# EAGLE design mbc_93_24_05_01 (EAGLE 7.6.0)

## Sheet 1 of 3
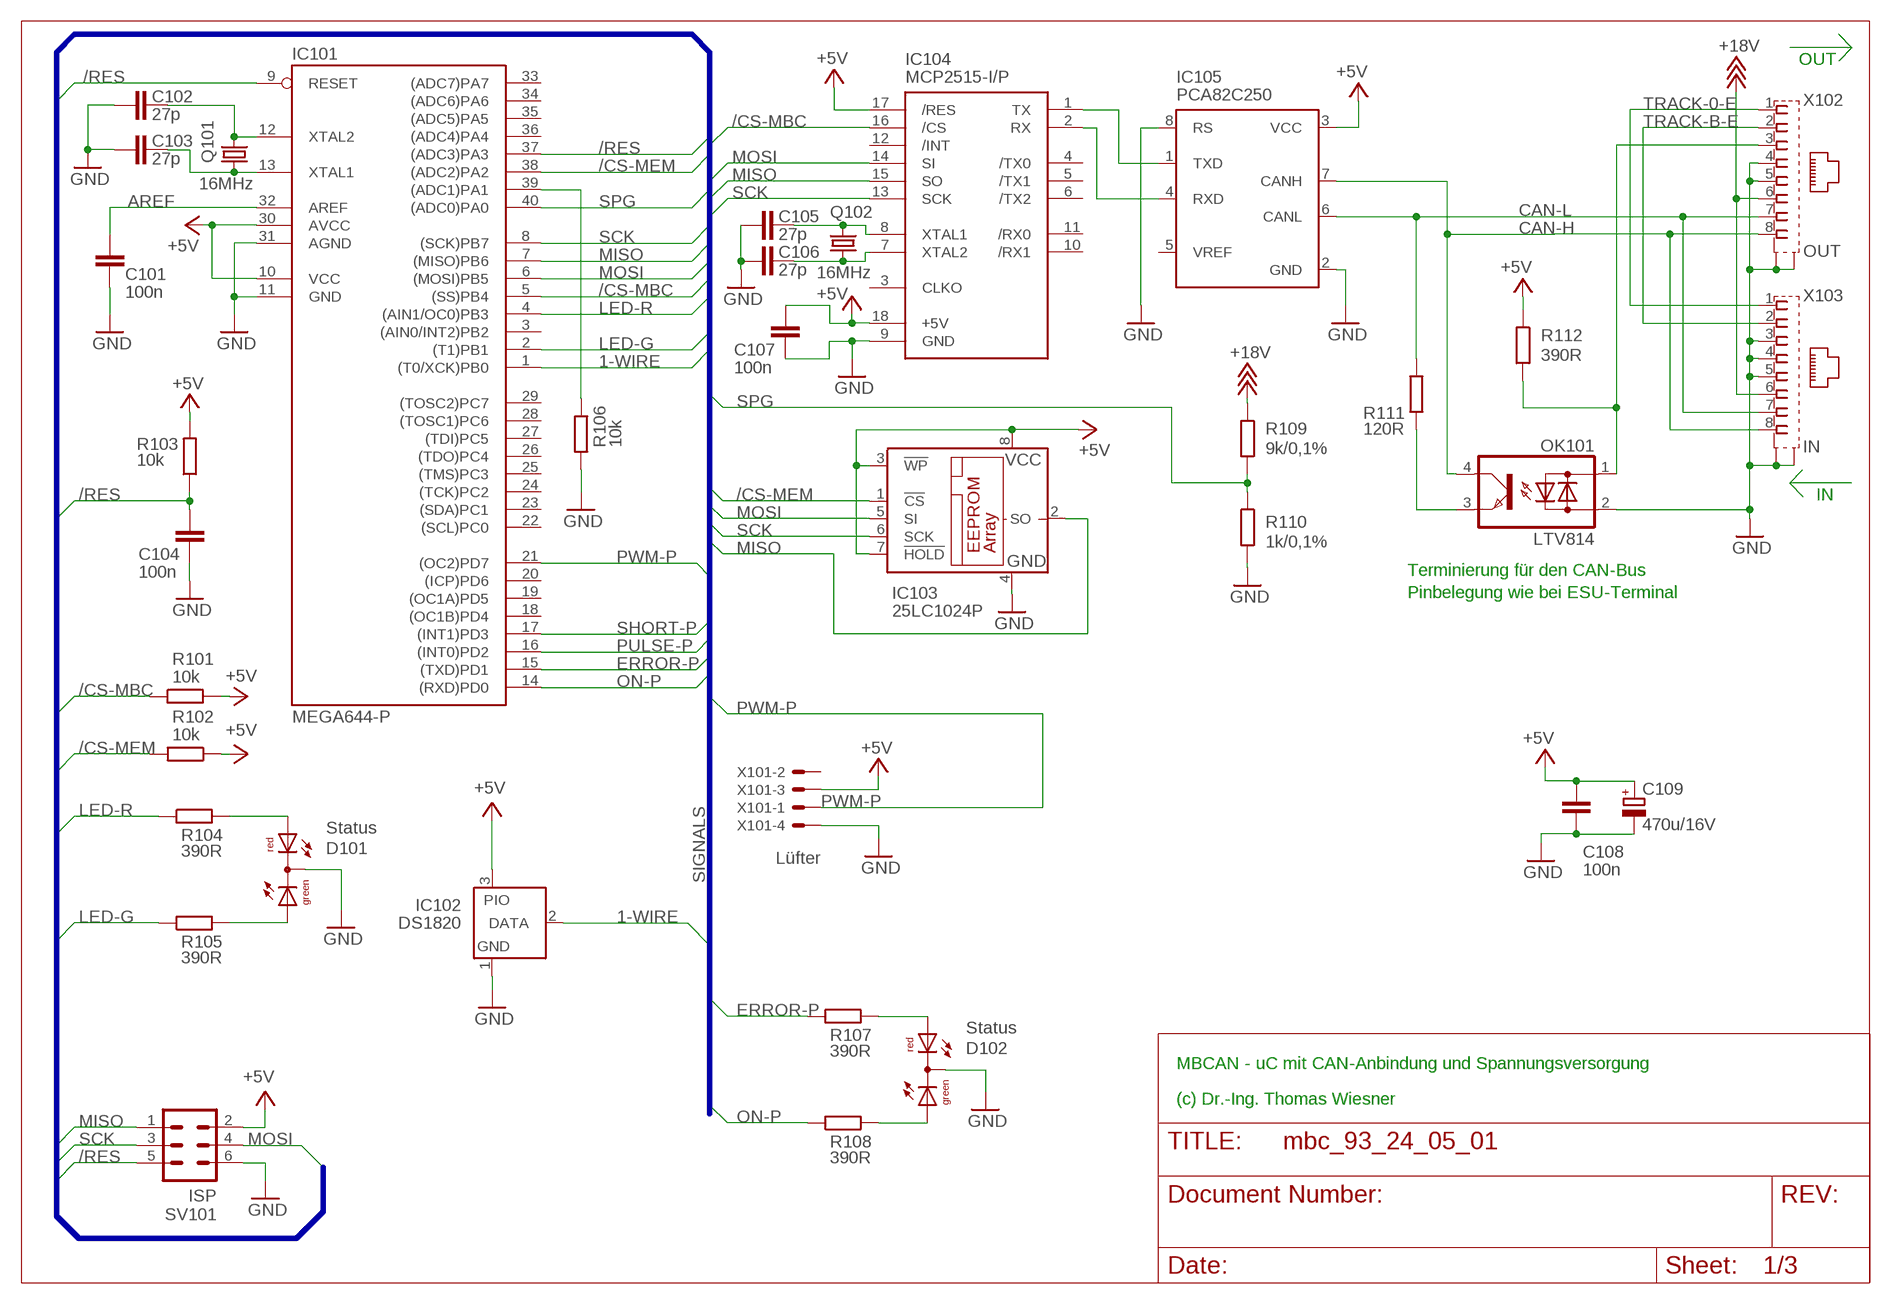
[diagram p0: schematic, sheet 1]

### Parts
C101  100n  C-EU025-025X050  [C025-025X050]
C102  27p  C-EU025-025X050  [C025-025X050]
C103  27p  C-EU025-025X050  [C025-025X050]
C104  100n  C-EU025-025X050  [C025-025X050]
C105  27p  C-EU025-025X050  [C025-025X050]
C106  27p  C-EU025-025X050  [C025-025X050]
C107  100n  C-EU025-025X050  [C025-025X050]
C108  100n  C-EU025-025X050  [C025-025X050]
C109  470u/16V  CPOL-EUE3.5-8  [E3,5-8]
D101  Status  DUOLED5MM  [DUOLED5MM]
D102  Status  DUOLED5MM  [DUOLED5MM]
IC101  MEGA644-P  MEGA323-P  [DIL40]
IC102  DS1820  DS2405  [TO92-]
IC103  25LC1024P  25LC040P  [DIL8]
IC104  MCP2515-I/P  MCP2510-I/P  [DIL18]
IC105  PCA82C250  [DIL08]
OK101  LTV814  PC814  [DIL04]
Q101  16MHz  CRYSTALHC49U-V  [HC49U-V]
Q102  16MHz  CRYSTALHC49U-V  [HC49U-V]
R101  10k  R-EU_0207/10  [0207/10]
R102  10k  R-EU_0207/10  [0207/10]
R103  10k  R-EU_0207/10  [0207/10]
R104  390R  R-EU_0207/10  [0207/10]
R105  390R  R-EU_0207/10  [0207/10]
R106  10k  R-EU_0207/10  [0207/10]
R107  390R  R-EU_0207/10  [0207/10]
R108  390R  R-EU_0207/10  [0207/10]
R109  9k/0,1%  R-EU_0207/10  [0207/10]
R110  1k/0,1%  R-EU_0207/10  [0207/10]
R111  120R  R-EU_0207/10  [0207/10]
R112  390R  R-EU_0207/10  [0207/10]
SV101  ISP  ML6  [ML6]
X101  Lüfter  22-23-2041  [22-23-2041]
X102  OUT  0446200002  [0446200002]
X103  IN  0446200002  [0446200002]

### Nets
1-WIRE: IC101.1((T0/XCK)PB0) IC102.2(DATA)
+5V: C107.1 C108.1 C109.+ IC101.10(VCC) IC101.30(AVCC) IC102.3(PIO) IC103.3(!WP) IC103.7(!HOLD) IC103.8(VCC) IC104.17(/RES) IC104.18(+5V) IC105.3(VCC) R101.2 R102.1 R103.2 R112.1 SV101.2 X101.3 ; also sheet 2,3
+18V: R109.1 X102.6 X103.6
/CS-MBC: IC101.5((SS)PB4) IC104.16(/CS) R101.1
/CS-MEM: IC101.38((ADC2)PA2) IC103.1(!CS) R102.2
/RES: C104.1 IC101.9(RESET) IC101.37((ADC3)PA3) R103.1 SV101.5
AREF: C101.1 IC101.32(AREF)
CAN-H: IC105.7(CANH) OK101.4(C) X102.8 X103.8
CAN-L: IC105.6(CANL) R111.2 X102.7 X103.7
ERROR-P: IC101.15((TXD)PD1) R107.1
GND: C101.2 C102.2 C103.2 C104.2 C105.2 C106.2 C107.2 C108.2 C109.- D101.K(C) D102.K(C) IC101.11(GND) IC101.31(AGND) IC102.1(GND) IC103.4(GND) IC104.9(GND) IC105.2(GND) IC105.8(RS) OK101.2(AC2) R106.1 R110.2 SV101.6 X101.4 X102.4 X102.5 X102.S@1(S1) X102.S@2(S2) X103.3 X103.4 X103.5 X103.S@1(S1) X103.S@2(S2) ; also sheet 2,3
LED-G: IC101.2((T1)PB1) R105.1
LED-R: IC101.4((AIN1/OC0)PB3) R104.1
MISO: IC101.7((MISO)PB6) IC103.2(SO) IC104.15(SO) SV101.1
MOSI: IC101.6((MOSI)PB5) IC103.5(SI) IC104.14(SI) SV101.4
N$1: C103.1 IC101.13(XTAL1) Q101.1
N$5: C102.1 IC101.12(XTAL2) Q101.2
N$6: C105.1 IC104.8(XTAL1) Q102.2
N$7: C106.1 IC104.7(XTAL2) Q102.1
N$9: IC101.39((ADC1)PA1) R106.2
N$23: D101.AR R104.2
N$27: D101.AG R105.2
N$29: IC104.1(TX) IC105.1(TXD)
N$30: IC104.2(RX) IC105.4(RXD)
N$32: OK101.3(E) R111.1
N$33: OK101.1(AC1) R112.2 X102.3
N$55: D102.AR R107.2
N$56: D102.AG R108.2
ON-P: IC101.14((RXD)PD0) R108.1 ; also sheet 2,3
PULSE-P: IC101.16((INT0)PD2) ; also sheet 2
PWM-P: IC101.21((OC2)PD7) X101.1
SCK: IC101.8((SCK)PB7) IC103.6(SCK) IC104.13(SCK) SV101.3
SHORT-P: IC101.17((INT1)PD3) ; also sheet 2,3
SPG: IC101.40((ADC0)PA0) R109.2 R110.1
TRACK-0-E: X102.1 X103.1 ; also sheet 2
TRACK-B-E: X102.2 X103.2 ; also sheet 2
Unconnected: IC101.3((AIN0/INT2)PB2) IC101.18((OC1B)PD4) IC101.19((OC1A)PD5) IC101.20((ICP)PD6) IC101.22((SCL)PC0) IC101.23((SDA)PC1) IC101.24((TCK)PC2) IC101.25((TMS)PC3) IC101.26((TDO)PC4) IC101.27((TDI)PC5) IC101.28((TOSC1)PC6) IC101.29((TOSC2)PC7) IC101.33((ADC7)PA7) IC101.34((ADC6)PA6) IC101.35((ADC5)PA5) IC101.36((ADC4)PA4) IC104.3(CLKO) IC104.4(/TX0) IC104.5(/TX1) IC104.6(/TX2) IC104.10(/RX1) IC104.11(/RX0) IC104.12(/INT) IC105.5(VREF) X101.2

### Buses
SIGNALS

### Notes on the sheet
- OUT
- IN
- Terminierung für den CAN-Bus
- Pinbelegung wie bei ESU-Terminal
- MBCAN - uC mit CAN-Anbindung und Spannungsversorgung
- (c) Dr.-Ing. Thomas Wiesner

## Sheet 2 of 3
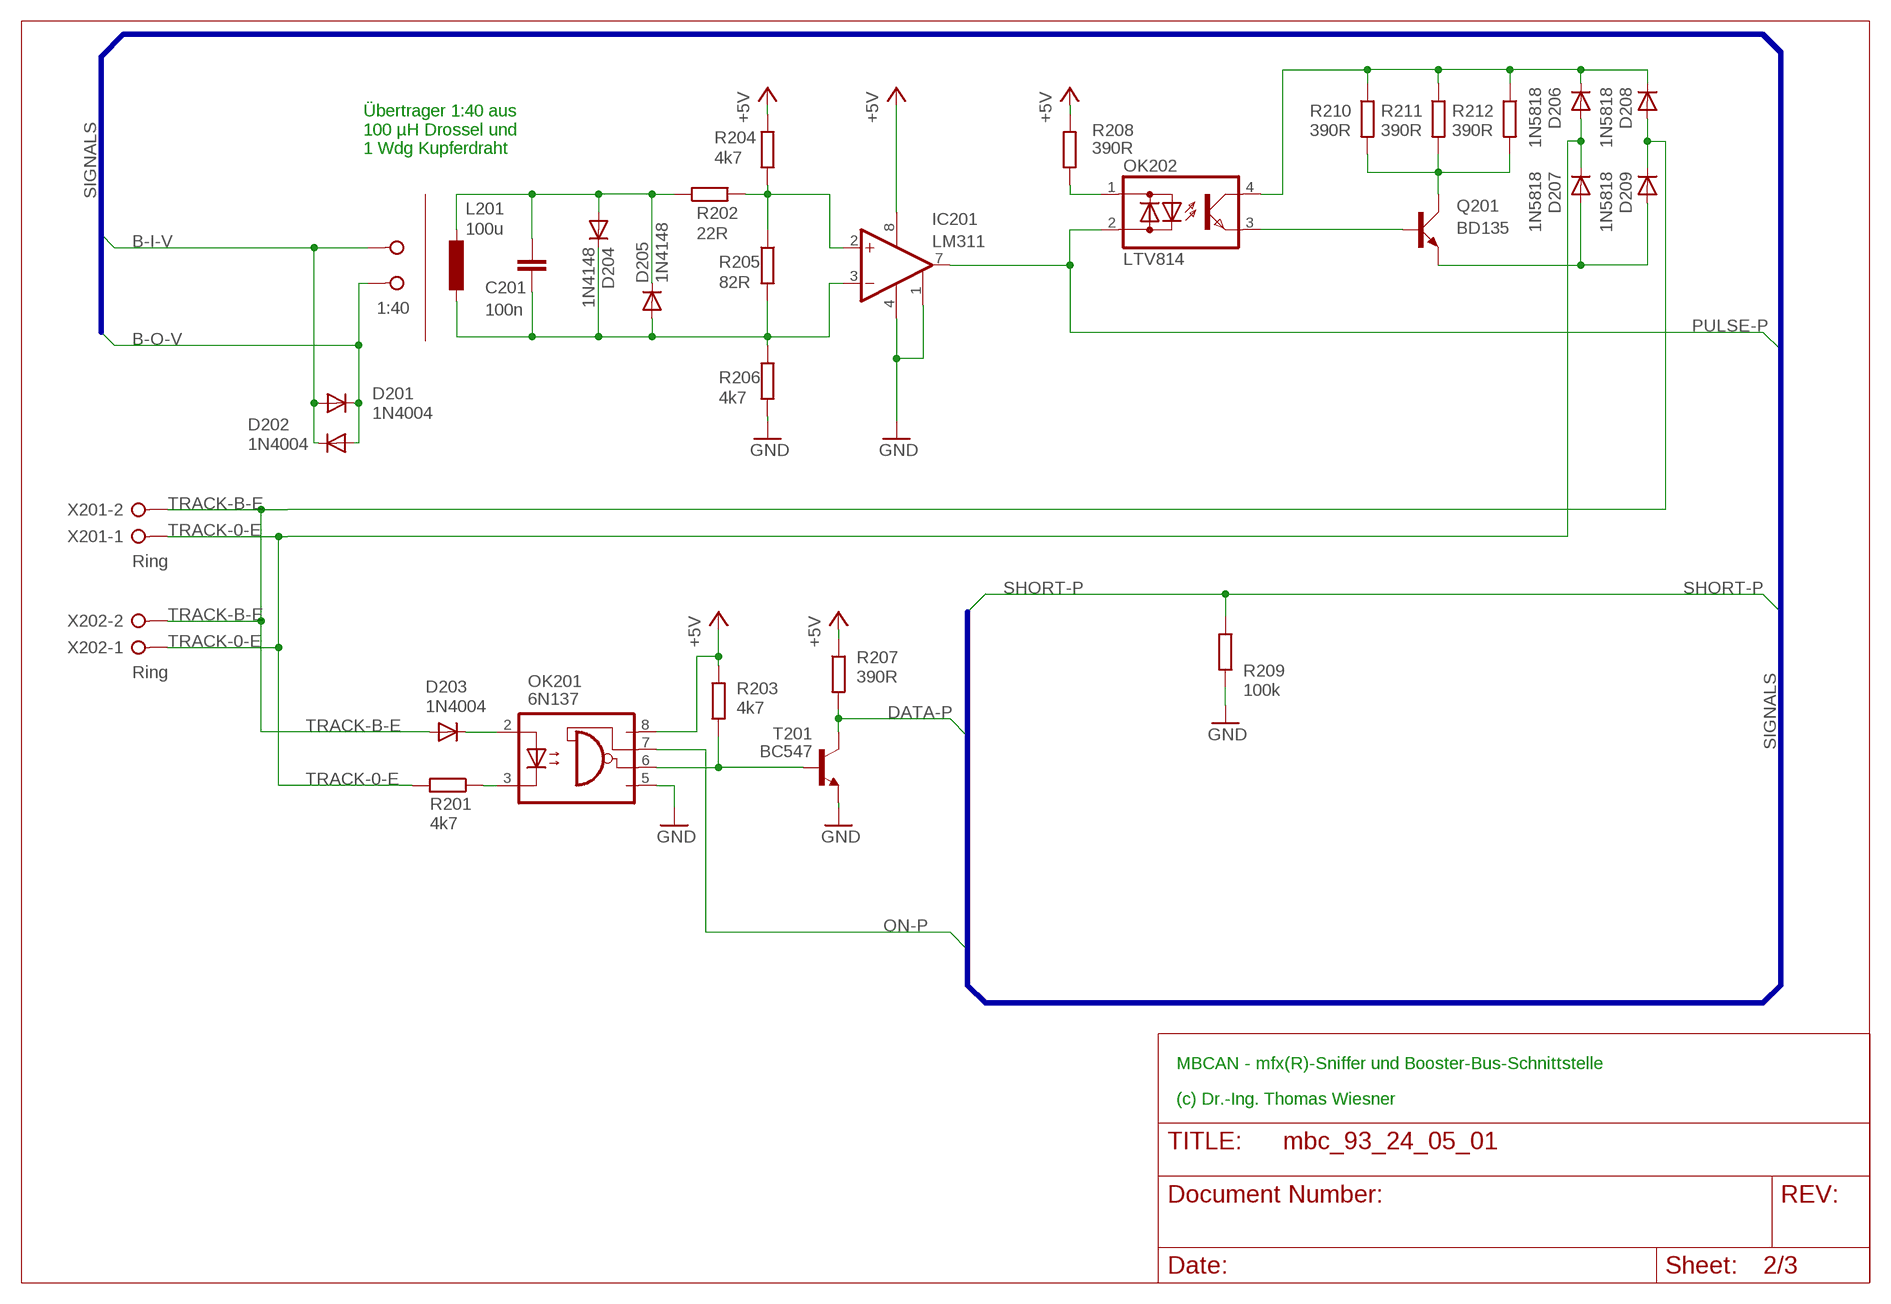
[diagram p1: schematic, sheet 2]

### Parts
C201  100n  C-EU025-025X050  [C025-025X050]
D201  1N4004  [DO41-10]
D202  1N4004  [DO41-10]
D203  1N4004  [DO41-10]
D204  1N4148  1N4148DO35-10  [DO35-10]
D205  1N4148  1N4148DO35-10  [DO35-10]
D206  1N5818  1N4004  [DO41-10]
D207  1N5818  1N4004  [DO41-10]
D208  1N5818  1N4004  [DO41-10]
D209  1N5818  1N4004  [DO41-10]
IC201  LM311  [DIL08]
L201  100u  L-EU6000-XXX-RC  [6000-XXXX-RC]
OK201  6N137  [DIL08]
OK202  LTV814  PC814  [DIL04]
Q201  BD135  BD139  [TO126AV]
R201  4k7  R-EU_0207/10  [0207/10]
R202  22R  R-EU_0207/10  [0207/10]
R203  4k7  R-EU_0207/10  [0207/10]
R204  4k7  R-EU_0207/10  [0207/10]
R205  82R  R-EU_0207/10  [0207/10]
R206  4k7  R-EU_0207/10  [0207/10]
R207  390R  R-EU_0207/10  [0207/10]
R208  390R  R-EU_0207/10  [0207/10]
R209  100k  R-EU_0207/10  [0207/10]
R210  390R  R-EU_0207/10  [0207/10]
R211  390R  R-EU_0207/10  [0207/10]
R212  390R  R-EU_0207/10  [0207/10]
T201  BC547  [TO92]
TP  1:40  W237-02P  [W237-132]
X201  Ring  W237-02P  [W237-132]
X202  Ring  W237-02P  [W237-132]

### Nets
+5V: IC201.8(V+) OK201.8(VCC) R203.1 R204.2 R207.1 R208.2 ; also sheet 1,3
B-I-V: D201.A D202.C TP.2 ; also sheet 3
B-O-V: D201.C D202.A TP.1 ; also sheet 3
DATA-P: R207.2 T201.3(C) ; also sheet 3
GND: IC201.1(EMIOUT) IC201.4(V-) OK201.5(GND) R206.2 R209.2 T201.1(E) ; also sheet 1,3
N$36: D206.C D208.C OK202.4(C) R210.1 R211.1 R212.1
N$37: D203.C OK201.2(A)
N$38: OK201.3(C) R201.1
N$39: C201.1 D204.A D205.C L201.1 R202.1
N$41: OK201.6(VO) R203.2 T201.2(B)
N$42: D207.A D209.A Q201.E
N$43: C201.2 D204.C D205.A IC201.3(-IN) L201.2 R205.2 R206.1
N$44: IC201.2(+IN) R202.2 R204.1 R205.1
N$45: OK202.3(E) Q201.B
N$46: Q201.C R210.2 R211.2 R212.2
N$50: OK202.1(AC1) R208.1
ON-P: OK201.7(VE) ; also sheet 1,3
PULSE-P: IC201.7(COLOUT) OK202.2(AC2) ; also sheet 1
SHORT-P: R209.1 ; also sheet 1,3
TRACK-0-E: D206.A D207.C R201.2 X201.1 X202.1 ; also sheet 1
TRACK-B-E: D203.A D208.A D209.C X201.2 X202.2 ; also sheet 1

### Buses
SIGNALS

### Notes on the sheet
- Übertrager 1:40 aus
  100 µH Drossel und 
  1 Wdg Kupferdraht
- MBCAN - mfx(R)-Sniffer und Booster-Bus-Schnittstelle
- (c) Dr.-Ing. Thomas Wiesner

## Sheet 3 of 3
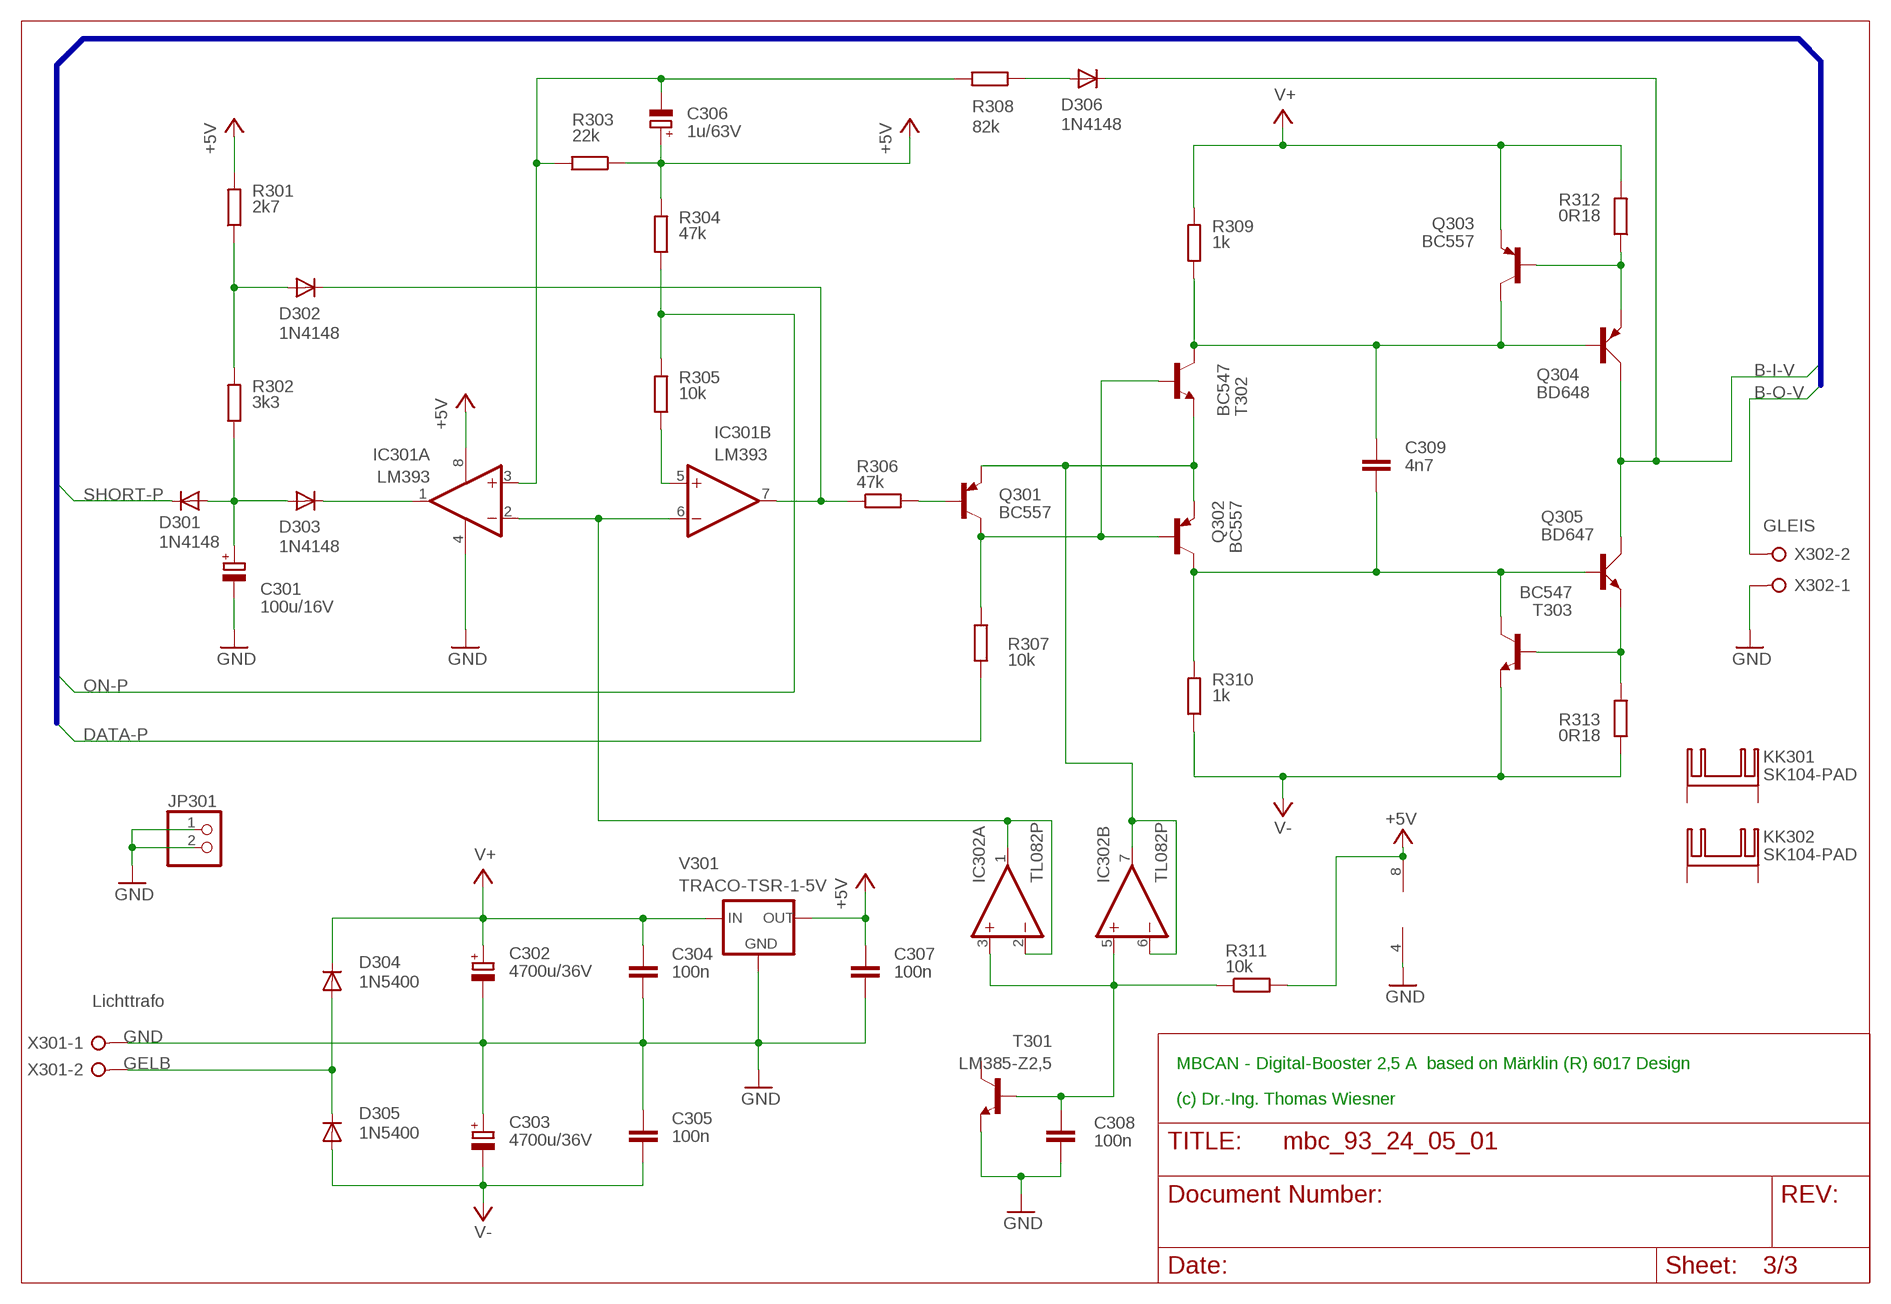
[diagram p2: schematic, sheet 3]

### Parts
C301  100u/16V  CPOL-EUE3.5-8  [E3,5-8]
C302  4700u/36V  CPOL-EUE7.5-16  [E7,5-16]
C303  4700u/36V  CPOL-EUE7.5-16  [E7,5-16]
C304  100n  C-EU025-024X044  [C025-024X044]
C305  100n  C-EU025-024X044  [C025-024X044]
C306  1u/63V  CPOL-EUE2.5-6  [E2,5-6]
C307  100n  C-EU025-024X044  [C025-024X044]
C308  100n  C-EU025-025X050  [C025-025X050]
C309  4n7  C-EU025-024X044  [C025-024X044]
D301  1N4148  1N4148DO35-7  [DO35-7]
D302  1N4148  1N4148DO35-7  [DO35-7]
D303  1N4148  1N4148DO35-7  [DO35-7]
D304  1N5400  [DO201-15]
D305  1N5400  [DO201-15]
D306  1N4148  1N4148DO35-7  [DO35-7]
IC301  LM393  [DIL08]
IC302  TL082P  [DIL08]
JP301  PINHD-1X2  [1X02]
KK301  SK104-PAD  [SK104-PAD]
KK302  SK104-PAD  [SK104-PAD]
Q301  BC557  [TO92]
Q302  BC557  [TO92]
Q303  BC557  [TO92]
Q304  BD648  TIP42C  [TO220AV]
Q305  BD647  TIP41C  [TO220AV]
R301  2k7  R-EU_0207/10  [0207/10]
R302  3k3  R-EU_0207/10  [0207/10]
R303  22k  R-EU_0207/10  [0207/10]
R304  47k  R-EU_0207/10  [0207/10]
R305  10k  R-EU_0207/10  [0207/10]
R306  47k  R-EU_0207/10  [0207/10]
R307  10k  R-EU_0207/10  [0207/10]
R308  82k  R-EU_0207/10  [0207/10]
R309  1k  R-EU_0207/10  [0207/10]
R310  1k  R-EU_0207/10  [0207/10]
R311  10k  R-EU_0207/10  [0207/10]
R312  0R18  R-EU_0414/15  [0414/15]
R313  0R18  R-EU_0414/15  [0414/15]
T301  LM385-Z2,5  BC547  [TO92]
T302  BC547  [TO92]
T303  BC547  [TO92]
V301  TRACO-TSR-1-5V  [TRACO-TSR-1]
X301  Lichttrafo  W237-02P  [W237-132]
X302  GLEIS  W237-02P  [W237-132]

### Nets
+5V: C306.+ C307.1 IC301.8(A:V+) IC302.8(P:V+) R301.2 R303.1 R304.2 R311.2 V301.OUT ; also sheet 1,2
B-I-V: D306.C Q304.C Q305.C ; also sheet 2
B-O-V: X302.2 ; also sheet 2
DATA-P: R307.1 ; also sheet 2
GELB: D304.A D305.C X301.2
GND: C301.- C302.- C303.+ C304.2 C305.1 C307.2 C308.2 IC301.4(A:V-) IC302.4(P:V-) JP301.1 JP301.2 T301.1(E) V301.GND X301.1 X302.1 ; also sheet 1,2
N$2: C309.1 Q303.3(C) Q304.B R309.1 T302.3(C)
N$3: Q303.2(B) Q304.E R312.1
N$4: Q305.E R313.2 T303.2(B)
N$8: C309.2 Q302.3(C) Q305.B R310.2 T303.3(C)
N$10: C308.1 IC302.3(A:+IN) IC302.5(B:+IN) R311.1 T301.2(B)
N$11: IC301.2(A:-IN) IC301.6(B:-IN) IC302.1(A:OUT) IC302.2(A:-IN)
N$15: IC301.5(B:+IN) R305.1
N$16: IC302.6(B:-IN) IC302.7(B:OUT) Q301.1(E) Q302.1(E) T302.1(E)
N$17: Q301.3(C) Q302.2(B) R307.2 T302.2(B)
N$18: Q301.2(B) R306.2
N$19: C306.- IC301.3(A:+IN) R303.2 R308.2
N$20: D306.A R308.1
N$22: D302.C IC301.7(B:COLOUT) R306.1
N$24: D303.C IC301.1(A:COLOUT)
N$25: C301.+ D301.A D303.A R302.1
N$26: D302.A R301.1 R302.2
ON-P: R304.1 R305.2 ; also sheet 1,2
SHORT-P: D301.C ; also sheet 1,2
V+: C302.+ C304.1 D304.C Q303.1(E) R309.2 R312.2 V301.IN
V-: C303.- C305.2 D305.A R310.1 R313.1 T303.1(E)
Unconnected: KK301.K1(K) KK301.K2(K) KK302.K1(K) KK302.K2(K) T301.3(C)

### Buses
B$1

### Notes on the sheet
- MBCAN - Digital-Booster 2,5 A  based on Märklin (R) 6017 Design
- (c) Dr.-Ing. Thomas Wiesner

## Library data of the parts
C101-C108 C201 C304 C305 C307-C309 = rcl:C-EU: CAPACITOR, European symbol
C109 C301-C303 C306 = rcl:CPOL-EU: POLARIZED CAPACITOR, European symbol
D101 D102 = led:DUOLED5MM: DUO LED 2 colors, 5 mm, round
D201-D203 D206-D209 = diode:1N4004: DIODE
D204 D205 D301-D303 D306 = diode:1N4148: DIODE
D304 D305 = diode:1N5400: DIODE
IC101 = atmel:MEGA323-P: MICROCONTROLLER 32 Kbytes FLASH 2 Kbytes SRAM 1 Kbytes EEPROM USART 8-channel 10 bit ADC Source: avr.lbr; OC_FARNELL: unknown; OC_NEWARK: unknown
IC102 = maxim:DS2405: Addressable Switch DALLAS Semiconductor; MF: DALLAS SEMICONDUCTOR; MPN: DS2405; OC_FARNELL: 1188025; OC_NEWARK: 06F4645
IC103 = microchip:25*: Serial EEPROM 4K/ 8K , SPI bus; MF: MICROCHIP; MPN: 25LC040/P; OC_FARNELL: 9758100; OC_NEWARK: 96K4091
IC104 = mbc:MCP2510: BASIC-CAN 2.0a Controller Stand-alone CAN controller von Microchip
IC105 = micro-philips:PCA82C250: CAN CONTROLLER INTERFACE; OC_FARNELL: 3692358; OC_NEWARK: unknown
IC201 = mbc:LM311: DC-Comparator Single
IC301 = mbc:LM393: DC-Comparator Dual
IC302 = linear:TL082: OP AMP Data sheet; DATA_SHEET: <a href="http://www.ti.com/lit/ds/symlink/tl084a.pdf"> Data sheet </a>
JP301 = pinhead:PINHD-1X2: PIN HEADER
KK301 KK302 = heatsink:SK104-PAD: HEATSINK
L201 = rcl:L-EU: INDUCTOR, European symbol
OK101 OK202 = optocoupler:PC814: SHARP OPTO COUPLER; OC_FARNELL: 9707662; OC_NEWARK: unknown
OK201 = optocoupler:6N137: MOTOROLA OPTO COUPLER; MPN: 6N137; OC_FARNELL: 1328376; OC_NEWARK: 52M1895
Q101 Q102 = crystal:CRYSTAL: CRYSTAL; OC_FARNELL: 1666969; OC_NEWARK: unknown
Q201 = transistor-power:BD139: NPN TRANSISTOR
Q301-Q303 = transistor-pnp:BC557: PNP Transistor
Q304 = transistor-power:TIP42C: PNP TRANSISTOR
Q305 = transistor-power:TIP41C: NPN TRANSISTOR
R101-R112 R201-R212 = resistor:R-EU_: RESISTOR, European symbol
R301-R313 = rcl:R-EU_: RESISTOR, European symbol
SV101 = con-ml:ML6: HARTING; OC_FARNELL: unknown; OC_NEWARK: unknown
T201 T301-T303 = transistor:BC547: NPN TRANSISTOR
TP X201 X202 X301 X302 = con-wago-508:W237-02P: WAGO SREW CLAMP; OC_FARNELL: unknown; OC_NEWARK: unknown
V301 = mbc:TRACO-TSR-1-5V: Spannungsregler Hersteller: TRACO Typ: TSR-1 5V: TSR 1-2450 Spg: 5V Strom: 1A Reichelt TSR 1-2450
X101 = con-molex:22-23-2041: .100" (2.54mm) Center Header - 4 Pin; MF: MOLEX; MPN: 22-23-2041; OC_FARNELL: 1462920; OC_NEWARK: 38C0355
X102 X103 = mbc:0446200002: RJ-45 INVERTED MODULAR JACK ASSEMBLY WITH RJ-11 KEEPOUT FEATURE Source: Data sheet MOLEX 0446200002 BUCHSE, RJ45, GESCHIRMT Source: Farnell; MF: MOLEX; MPN: 0446200002; OC_FARNELL: 9251910

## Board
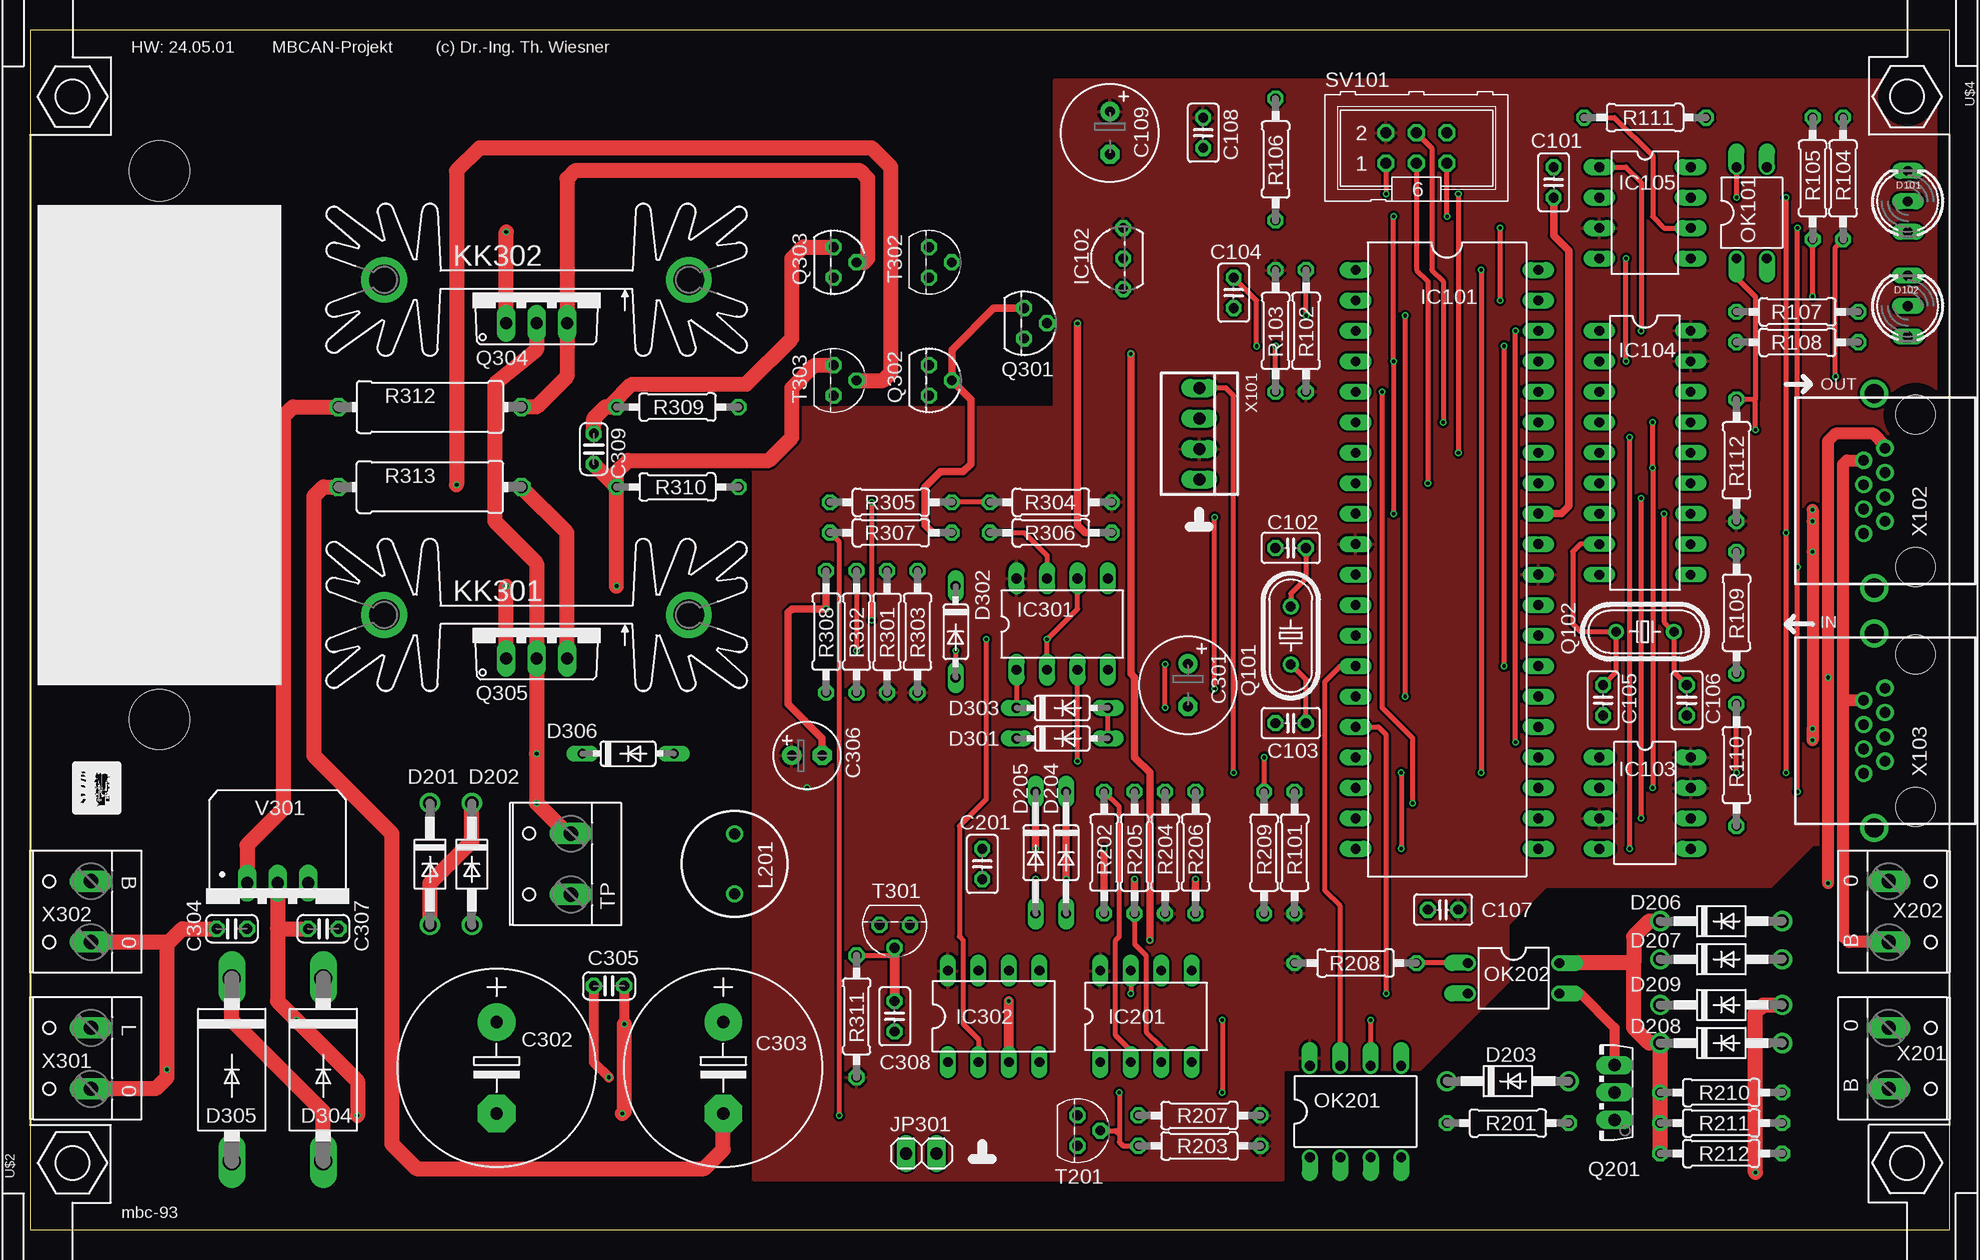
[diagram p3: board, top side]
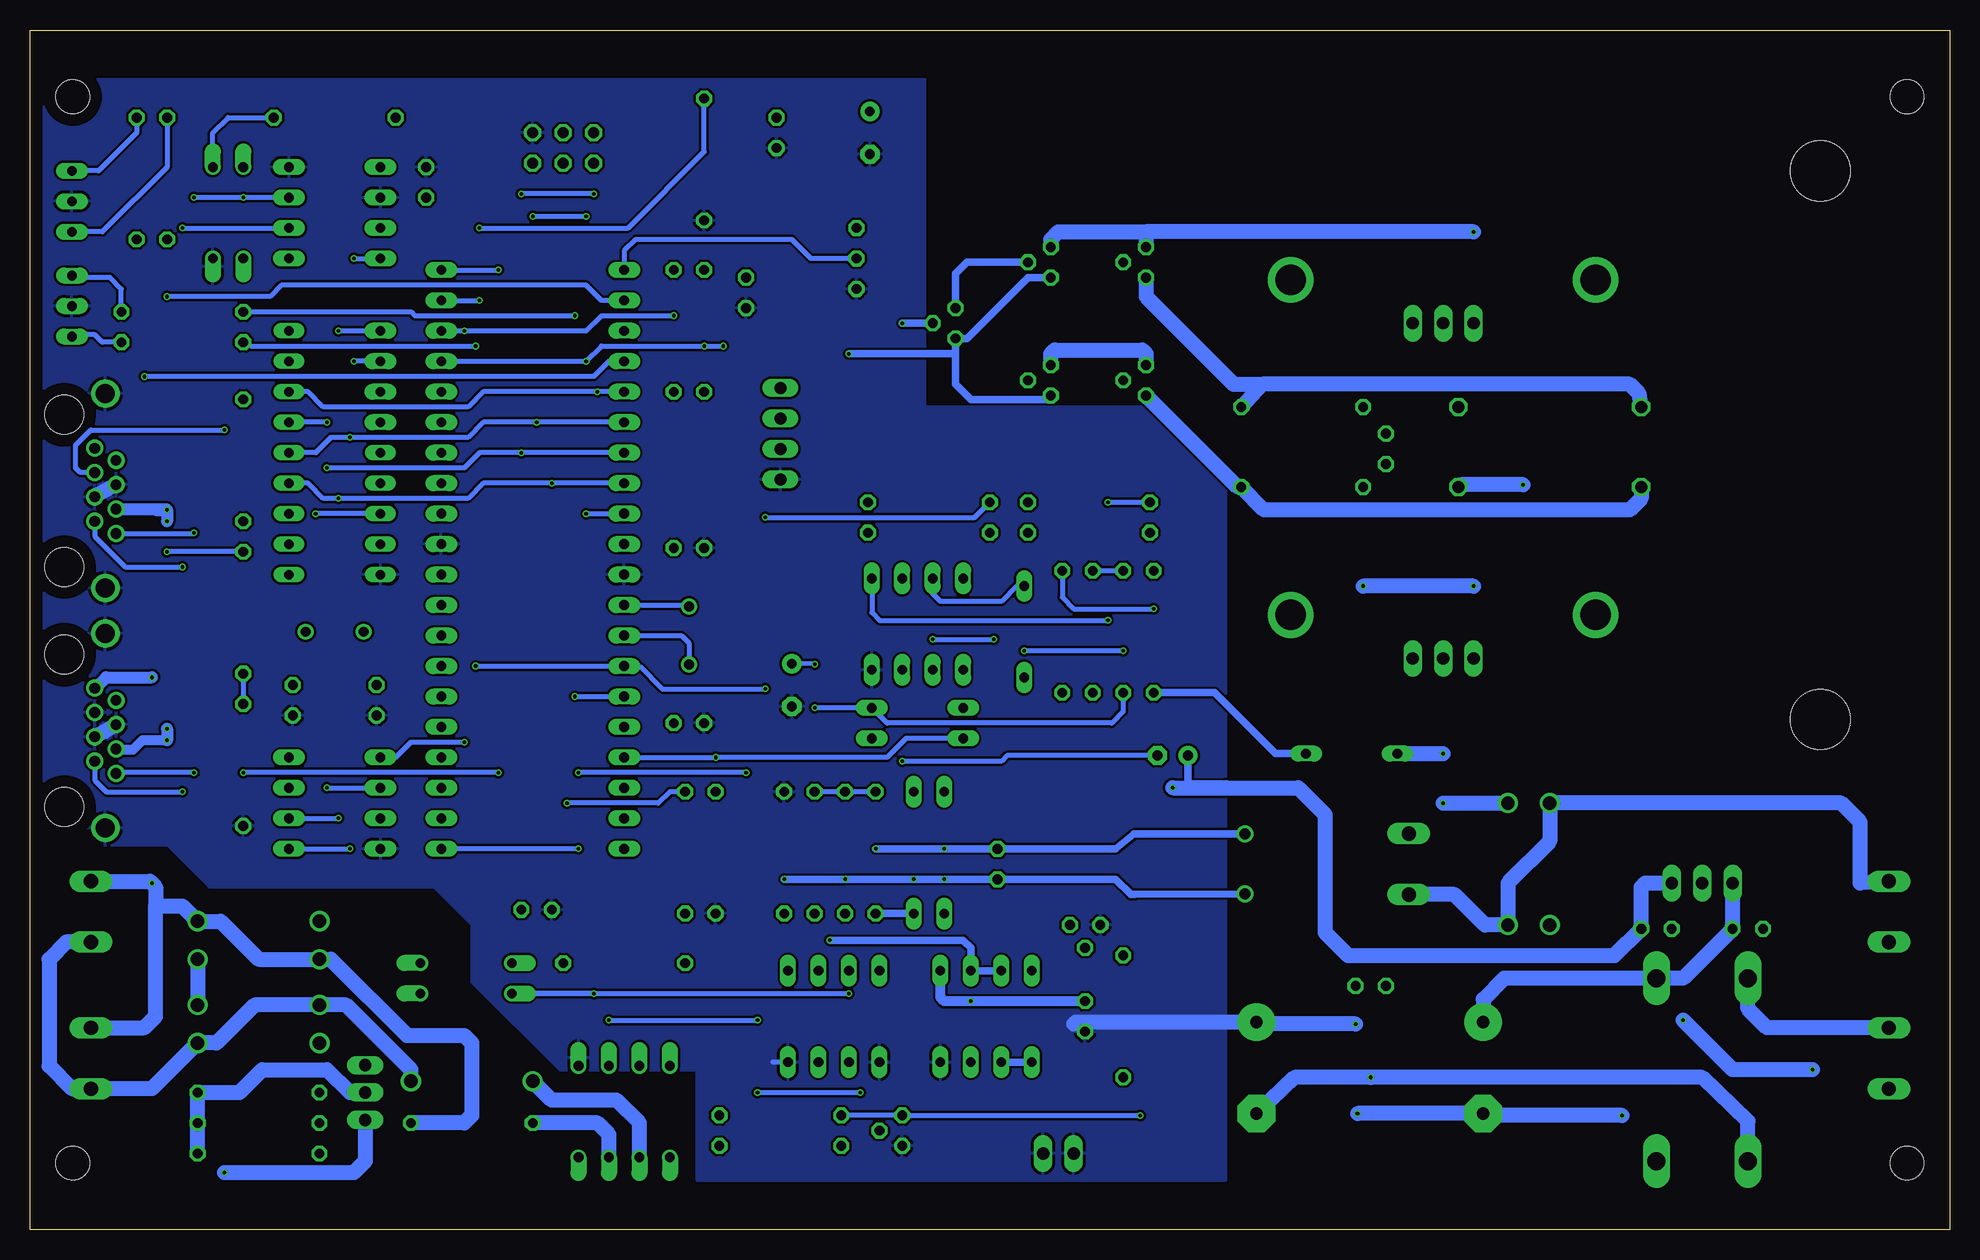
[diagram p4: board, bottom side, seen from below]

Size 160.02 x 100.01 mm. Coordinates in mm from the lower left corner, seen from the top.
Outline: 0,0 160.02,0 160.02,100.01 0,100.01 0,0
Copper layers (1*16): Top 0.035mm / dielectric 1.5mm / Bottom 0.035mm
Design rules "default *": minimum track width 10mil, minimum drill 0.3mm, track to track 8mil, track to pad 8mil, pad to pad 8mil, via to via 8mil, smd to smd 8mil, copper to edge 40mil, drill to drill 8mil, minimum pad ring 10mil, minimum via ring 0.125mm, stop-mask expansion 4mil, vias tented up to drill 0mil, thermal gap 10mil
Holes 5 mm at 10.79,88.27 10.79,42.55

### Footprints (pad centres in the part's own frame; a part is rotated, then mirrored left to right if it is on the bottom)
C025-025X050 = drill 0.813 octagon: 1 -1.27,0; 2 1.27,0
E3,5-8 = drill 0.813 pad 1.6: + -1.778,0 | drill 0.813 pad 1.6 octagon: - 1.778,0
E7,5-16 = drill 1.016 pad 3.15: + -3.81,0 | drill 1.016 pad 3.15 octagon: - 3.81,0
C025-024X044 = drill 0.813 octagon: 1 -1.27,0; 2 1.27,0
E2,5-6 = drill 0.813 pad 1.6: + -1.27,0 | drill 0.813 pad 1.6 octagon: - 1.27,0
DUOLED5MM = drill 0.813 long: AG -2.54,0; AR 2.54,0; K 0,0
DO41-10 = drill 1.118: A 5.08,0; C -5.08,0
DO35-10 = drill 0.813 long: A 5.08,0; C -5.08,0
DO35-7 = drill 0.813 long: A 3.81,0; C -3.81,0
DO201-15 = drill 1.499 long: A 7.62,0; C -7.62,0
DIL40 = drill 0.813 long: 1 -24.13,-7.62; 2 -21.59,-7.62; 3 -19.05,-7.62; 4 -16.51,-7.62; 5 -13.97,-7.62; 6 -11.43,-7.62; 7 -8.89,-7.62; 8 -6.35,-7.62; 9 -3.81,-7.62; 10 -1.27,-7.62; 11 1.27,-7.62; 12 3.81,-7.62; 13 6.35,-7.62; 14 8.89,-7.62; 15 11.43,-7.62; 16 13.97,-7.62; 17 16.51,-7.62; 18 19.05,-7.62; 19 21.59,-7.62; 20 24.13,-7.62; 21 24.13,7.62; 22 21.59,7.62; 23 19.05,7.62; 24 16.51,7.62; 25 13.97,7.62; 26 11.43,7.62; 27 8.89,7.62; 28 6.35,7.62; 29 3.81,7.62; 30 1.27,7.62; 31 -1.27,7.62; 32 -3.81,7.62; 33 -6.35,7.62; 34 -8.89,7.62; 35 -11.43,7.62; 36 -13.97,7.62; 37 -16.51,7.62; 38 -19.05,7.62; 39 -21.59,7.62; 40 -24.13,7.62
TO92- = drill 0.813 octagon: 1 -2.54,0; 2 0,0; 3 2.54,0
DIL8 = drill 0.813 long: 1 -3.81,-3.81; 2 -1.27,-3.81; 3 1.27,-3.81; 4 3.81,-3.81; 5 3.81,3.81; 6 1.27,3.81; 7 -1.27,3.81; 8 -3.81,3.81
DIL18 = drill 0.813 long: 1 -10.16,-3.81; 2 -7.62,-3.81; 3 -5.08,-3.81; 4 -2.54,-3.81 | drill 0.8 long: 5 0,-3.81; 6 2.54,-3.81; 7 5.08,-3.81; 8 7.62,-3.81; 9 10.16,-3.81; 10 10.16,3.81; 11 7.62,3.81; 12 5.08,3.81; 13 2.54,3.81; 14 0,3.81; 15 -2.54,3.81; 16 -5.08,3.81; 17 -7.62,3.81; 18 -10.16,3.81
DIL08 = drill 0.813 long: 1 -3.81,-3.81; 2 -1.27,-3.81; 3 1.27,-3.81; 4 3.81,-3.81; 5 3.81,3.81; 6 1.27,3.81; 7 -1.27,3.81; 8 -3.81,3.81
DIL08' = drill 0.813 pad 1.27 long: 1 -3.81,-3.81; 2 -1.27,-3.81; 3 1.27,-3.81; 4 3.81,-3.81; 5 3.81,3.81; 6 1.27,3.81; 7 -1.27,3.81; 8 -3.81,3.81
1X02 = drill 1.016 long: 1 -1.27,0; 2 1.27,0
SK104-PAD = drill 2.54 pad 3.81: K1 -12.7,-0.762; K2 12.7,-0.762
6000-XXXX-RC = drill 0.9 pad 1.422: 1 -2.5,0; 2 2.5,0
DIL04 = drill 0.813 offset: 1 -1.27,-3.81; 2 1.27,-3.81; 3 1.27,3.81; 4 -1.27,3.81
DIL08'' = drill 0.813 offset: 1 -3.81,-3.81; 2 -1.27,-3.81; 3 1.27,-3.81; 4 3.81,-3.81; 5 3.81,3.81; 6 1.27,3.81; 7 -1.27,3.81; 8 -3.81,3.81
HC49U-V = drill 0.813: 1 -2.413,0; 2 2.413,0
TO126AV = drill 1.016 long: B 2.286,-1.27; C 0,-1.27; E -2.286,-1.27
TO92 = drill 0.813 octagon: 1 1.27,0; 2 0,1.905; 3 -1.27,0
TO220AV = drill 1.016 long: B -2.54,-2.54; C 0,-2.54; E 2.54,-2.54
0207/10 = drill 0.813 octagon: 1 -5.08,0; 2 5.08,0
0414/15 = drill 1.016 octagon: 1 -7.62,0; 2 7.62,0
ML6 = drill 0.914 octagon: 1 -2.54,-1.27; 2 -2.54,1.27; 3 0,-1.27; 4 0,1.27; 5 2.54,-1.27; 6 2.54,1.27
W237-132 = drill 1.194 long: 1 -2.54,-0.635; 2 2.54,-0.635
FPH = hole 2.794: 3.556,44.45; 3.556,-44.45
TRACO-TSR-1 = drill 1.016 long: GND 0,2.54; IN -2.54,2.54; OUT 2.54,2.54
22-23-2041 = drill 1 long: 1 -3.81,0; 2 -1.27,0; 3 1.27,0; 4 3.81,0
0446200002 = drill 0.889 pad 1.422: 1 3.556,2.54; 2 2.54,4.318; 3 1.524,2.54; 4 0.508,4.318; 5 -0.508,2.54; 6 -1.524,4.318; 7 -2.54,2.54; 8 -3.556,4.318 | drill 1.575 pad 2.286: S@1 -8.103,3.429; S@2 8.103,3.429 | hole 3.251: 6.35,0; -6.35,0

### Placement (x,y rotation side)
C101  127,87.31 90 top
C102  105.09,56.83 180 top
C103  105.09,42.23 180 top
C104  100.33,78.11 270 top
C105  131.13,44.13 270 top
C106  138.11,44.13 270 top
C107  117.79,26.67 180 top
C108  97.79,91.44 270 top
C109  90.01,91.44 270 top
C201  79.38,30.48 270 top
C301  96.52,45.4 270 top
C302  38.89,13.49 270 top
C303  57.78,13.49 270 top
C304  16.83,25.08 180 top
C305  48.26,20.32 180 top
C306  64.77,39.53 0 top
C307  24.45,25.08 180 top
C308  72.07,17.78 270 top
C309  46.99,65.09 270 top
D101  156.53,85.72 90 top
D102  156.53,76.99 90 top
D201  33.34,30.48 270 top
D202  36.83,30.48 270 top
D203  123.19,12.38 0 top
D204  86.36,31.43 270 top
D205  83.82,31.43 270 top
D206  140.97,25.72 0 top
D207  140.97,22.54 0 top
D208  140.97,15.56 0 top
D209  140.97,18.73 0 top
D301  86.04,40.96 0 top
D302  77.15,49.85 270 top
D303  86.04,43.5 0 top
D304  24.45,13.34 270 top
D305  16.83,13.34 270 top
D306  49.85,39.69 0 top
IC101  118.11,55.88 270 top
IC102  91.12,80.96 90 top
IC103  134.62,35.56 270 top
IC104  134.62,64.77 270 top
IC105  134.62,84.77 270 top
IC201  93.03,17.78 0 top
IC301  86.04,50.48 0 top
IC302  TL082P  [DIL08']  80.33,17.78 0 top
JP301  74.3,6.35 0 top
KK301  42.23,50.48 180 top
KK302  42.23,78.42 180 top
L201  58.74,30.48 270 top
OK101  143.51,84.77 0 top
OK201  6N137  [DIL08'']  110.49,9.84 0 top
OK202  123.67,20.95 270 top
Q101  105.09,49.53 90 top
Q102  134.62,49.85 180 top
Q201  130.81,11.43 90 top
Q301  82.87,75.56 270 top
Q302  74.93,70.8 270 top
Q303  66.99,80.64 270 top
Q304  42.23,78.11 0 top
Q305  42.23,50.16 0 top
R101  105.41,31.43 270 top
R102  106.36,74.93 90 top
R103  103.82,74.93 90 top
R104  151.13,87.63 90 top
R105  148.59,87.63 90 top
R106  103.82,89.22 90 top
R107  147.32,76.52 0 top
R108  147.32,73.98 0 top
R109  142.24,51.44 270 top
R110  142.24,38.73 270 top
R111  134.62,92.71 180 top
R112  142.24,64.14 90 top
R201  123.19,8.89 0 top
R202  89.53,31.43 90 top
R203  97.47,6.99 180 top
R204  94.61,31.43 270 top
R205  92.08,31.43 270 top
R206  97.16,31.43 90 top
R207  97.47,9.53 180 top
R208  110.49,22.23 180 top
R209  102.87,31.43 270 top
R210  140.97,11.43 0 top
R211  140.97,8.89 0 top
R212  140.97,6.35 0 top
R301  71.44,49.85 270 top
R302  68.9,49.85 90 top
R303  73.98,49.85 90 top
R304  85.09,60.64 0 top
R305  71.75,60.64 0 top
R306  85.09,58.1 0 top
R307  71.75,58.1 0 top
R308  66.36,49.85 90 top
R309  53.98,68.58 0 top
R310  53.98,61.91 180 top
R311  68.9,17.78 270 top
R312  33.34,68.58 180 top
R313  33.34,61.91 0 top
SV101  115.57,90.17 0 top
T201  87.31,8.26 270 top
T301  72.07,25.4 180 top
T302  74.93,80.64 270 top
T303  66.99,70.8 270 top
TP  44.45,30.48 90 top
U$2  [FPH]  0,50.01 0 top
U$4  [FPH]  160.02,50.01 180 top
V301  20.64,26.35 0 top
X101  97.47,66.36 270 top
X102  157.16,61.59 90 top
X103  157.16,41.59 90 top
X201  155.57,14.29 270 top
X202  155.57,26.51 270 top
X301  4.45,14.29 90 top
X302  4.45,26.51 90 top

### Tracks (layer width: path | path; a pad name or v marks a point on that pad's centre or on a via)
1-WIRE
  Bottom 0.406: IC102.2 94.93,80.96 96.52,82.55 109.54,82.55 110.49,81.6 IC101.1
+5V  (via drill 0.3)
  Bottom 0.61: C306.+ 63.5,37.15 60.64,37.15 60.33,36.83
  Bottom 1.27: V301.OUT 25.4,28.89 25.72,28.57 C307.1 27.94,22.86 50.16,22.86 52.07,24.77 52.07,34.61 54.29,36.83 60.33,36.83 v64.77,36.83
  pour Top: 85.41,95.89 160.02,95.89 160.02,32.07 148.59,32.07 145.1,28.57 126.36,28.57 123.19,25.4 123.19,20.64 115.89,13.34 104.46,13.34 104.46,4.13 60.33,4.13 60.33,68.58 85.41,68.58
+18V  (via drill 0.3)
  Top 1.016: v148.59,60.01 v148.59,59.05 v148.59,56.52 v148.59,40.8 v148.59,41.75
  Bottom 0.406: R109.1 v148.59,56.52
  Bottom 0.813: v148.59,40.8 150.65,40.8 151.45,40.01 152.78,40.01 X103.6
  Bottom 1.016: X102.6 148.65,60.07 v148.59,60.01 | v148.59,41.75 v148.59,40.8 | 149.54,60.01 v148.59,60.01 | v148.59,60.01 v148.59,59.05
/CS-MBC  (via drill 0.3)
  Top 0.406: v115.25,35.56 115.25,40.96 112.71,43.5 v112.71,69.85
  Bottom 0.406: IC101.5 v112.71,69.85 122.24,69.85 123.51,68.58 135.57,68.58 136.84,69.85 IC104.16 | R101.1 106.68,36.51 107.63,35.56 v115.25,35.56
/CS-MEM  (via drill 0.3)
  Top 0.406: v106.36,76.2 R102.2 | v123.83,40.64 v123.83,74.93
  Bottom 0.406: IC101.38 v123.83,74.93 113.67,74.93 112.39,76.2 v106.36,76.2 | IC103.1 129.54,39.37 128.27,40.64 v123.83,40.64
/RES  (via drill 0.3)
  Top 0.406: v113.67,59.69 v113.67,72.39 v113.67,84.45 | v118.11,84.45 SV101.5 | v102.23,73.66 102.23,77.47 C104.1 | R103.1 v103.82,73.66
  Bottom 0.406: IC101.37 v113.67,72.39 112.39,73.66 v103.82,73.66 v102.23,73.66 | v113.67,59.69 IC101.9 | v113.67,84.45 v118.11,84.45
AREF
  Top 0.61: C101.1 127,82.87 128.27,81.6 128.27,60.33 127.64,59.69 IC101.32
B-I-V  (via drill 0.3)
  Top 1.27: TP.2 44.77,33.02 v42.23,35.56 v42.23,39.69 Q305.C 42.23,55.56 38.73,59.05 38.73,70.48 42.23,73.34 Q304.C | D201.A 33.34,28.89 36.83,32.38 D202.C
  Bottom 1.27: v42.23,35.56 D202.C | D306.C v42.23,39.69
B-O-V
  Bottom 1.27: X302.2 7.46,28.89 7.46,33.97 9.05,35.56 D201.C 33.34,32.38 36.83,28.89 D202.A 38.73,25.4 41.27,27.94 TP.1
CAN-H  (via drill 0.3)
  Top 0.406: v146.37,86.04 v146.37,58.1 v146.37,38.1 | OK101.4 v142.24,86.04
  Bottom 0.406: IC105.7 v142.24,86.04 v146.37,86.04 | v146.37,38.1 152.78,38.1 X103.8 | X102.8 146.43,58.04 v146.37,58.1
CAN-L  (via drill 0.3)
  Top 0.406: v147.32,36.51 v147.32,55.24 v147.32,83.5 | R111.2 132.08,92.71 135.25,89.53 135.25,84.45 136.21,83.5 IC105.6
  Bottom 0.406: X103.7 154.62,37.47 153.67,36.51 v147.32,36.51 | v147.32,83.5 IC105.6 | X102.7 154.62,57.78 152.08,55.24 v147.32,55.24
DATA-P  (via drill 0.3)
  Top 0.406: v67.47,9.53 67.47,57.31 R307.1
  Bottom 0.406: v67.47,9.53 T201.3 R207.2
ERROR-P  (via drill 0.3)
  Top 0.406: v114.62,76.2 v114.62,44.45
  Bottom 0.406: R107.1 128.27,76.52 127.95,76.2 v114.62,76.2 | v114.62,44.45 IC101.15
GELB
  Top 1.27: D304.A 24.45,9.84 16.83,17.46 D305.C
  Bottom 1.27: X301.2 15.24,16.83 16.83,18.41 D305.C
GND  (via drill 0.3)
  Top 0.813: C305.1 v49.53,17.14
  Top 1.27: 11.43,23.81 v11.43,13.34 11.43,12.7 10.48,11.75 X301.1 | 11.43,23.81 12.7,25.08 C304.2 | X302.1 11.27,23.97 11.43,23.81 | V301.GND 20.64,25.08 | 20.64,25.08 20.64,19.05 v22.23,17.46 27.3,12.38 v27.3,9.53 | 20.64,25.08 C307.2 | v49.53,17.14 49.53,9.84 v49.37,9.68
  Bottom 0.406: IC201.4 98.11,13.97
  Bottom 0.61: C302.- 38.73,9.53
  Bottom 1.27: X102.4 154.59,61.15 154.62,61.12 154.59,61.12 X102.5 | X103.4 153.92,41.47 X103.5 | C302.- v49.37,9.68 | v49.53,17.14 57.47,17.14 C303.+ 72.87,17.3 73.03,17.14 | v27.3,9.53 38.73,9.53 | v11.43,13.34 18.1,13.34 v22.23,17.46
  pour Bottom: 160.02,95.89 160.02,32.07 148.59,32.07 145.1,28.57 126.36,28.57 123.19,25.4 123.19,20.64 115.89,13.34 104.46,13.34 104.46,4.13 60.33,4.13 60.33,68.58 85.41,68.58 85.41,95.89
LED-G  (via drill 0.3)
  Top 0.406: v148.59,77.79 R105.1
  Bottom 0.406: IC101.2 112.39,77.47 113.67,78.74 139.06,78.74 140.02,77.79 v148.59,77.79
LED-R  (via drill 0.3)
  Top 0.406: v150.5,71.12 150.5,81.92 R104.1
  Bottom 0.406: IC101.4 111.76,72.39 113.03,71.12 v150.5,71.12
MISO  (via drill 0.3)
  Top 0.406: v135.25,67.31 v135.25,63.5 v135.25,36.83 | SV101.1 v113.03,86.36 | v119.06,86.36 v119.06,64.77
  Bottom 0.406: IC101.7 v119.06,64.77 122.56,64.77 123.83,63.5 v135.25,63.5 | v135.25,67.31 IC104.15 | v113.03,86.36 v119.06,86.36 | v135.25,36.83 IC103.2
MOSI  (via drill 0.3)
  Top 0.406: SV101.4 116.84,90.17 116.84,80.01 117.79,79.06 v117.79,67.31 | v133.35,31.75 v133.35,66.04
  Bottom 0.406: IC101.6 v117.79,67.31 122.24,67.31 123.51,66.04 v133.35,66.04 134.94,66.04 136.21,64.77 IC104.14 | IC103.5 v133.35,31.75
N$1
  Top 0.406: C103.1 106.36,45.85 Q101.1
  Bottom 0.406: IC101.13 105.73,49.53 105.09,48.9 Q101.1
N$2  (via drill 0.3)
  Top 1.27: 47.05,67.25 46.99,67.31 | 46.99,67.31 46.99,67.63 47.94,68.58 R309.1 48.42,68.74 50.16,70.48 59.69,70.48 63.5,74.3 63.5,80.96 64.45,81.92 Q303.3 | C309.1 46.99,67.31 | Q304.B v39.69,83.19
  Bottom 1.27: T302.3 74.93,82.55 74.3,83.19 66.99,83.19 | 66.99,83.19 Q303.3 66.99,82.55 | v39.69,83.19 66.99,83.19
N$3
  Top 1.27: Q303.2 69.53,80.64 69.85,80.96 69.85,87.63 69.22,88.27 45.4,88.27 44.77,87.63 Q304.E 44.77,71.12 42.23,68.58 R312.1
N$4  (via drill 0.3)
  Top 1.27: T303.2 71.12,70.8 71.75,71.44 71.75,88.58 70.17,90.17 37.47,90.17 35.56,88.27 v35.56,62.1 | Q305.E 44.77,58.1 R313.2
  Bottom 1.27: v35.56,62.1 40.77,62.1 R313.2
N$5
  Top 0.406: C102.1 106.36,54.29 105.09,53.02 Q101.2
  Bottom 0.406: IC101.12 105.22,52.07 Q101.2
N$6
  Top 0.406: C105.1 132.21,46.48 Q102.2 129.22,49.85 128.59,50.48 128.59,56.52 129.22,57.15 IC104.8
N$7  (via drill 0.3)
  Top 0.406: C106.1 137.03,46.48 Q102.1 136.21,50.67 v136.21,59.69
  Bottom 0.406: IC104.7 v136.21,59.69
N$8  (via drill 0.3)
  Top 1.27: C309.2 R310.2 | R310.2 48.9,63.18 49.85,64.14 61.59,64.14 63.5,66.04 63.5,70.17 65.41,72.07 T303.3 | Q305.B v39.69,53.66 | v48.9,53.66 R310.2
  Bottom 1.27: Q302.3 74.93,73.03 74.61,73.34 67.31,73.34 66.99,73.03 T303.3 | v39.69,53.66 v48.9,53.66
N$9  (via drill 0.3)
  Top 0.406: v122.56,77.47 v122.56,83.5
  Bottom 0.406: IC101.39 v122.56,77.47 | v122.56,83.5 110.17,83.5 103.82,89.85 R106.2
N$10  (via drill 0.3)
  Top 0.406: R311.1 72.07,22.86 72.07,22.54
  Top 0.813: T301.2 72.07,22.54 C308.1 | IC302.3 v81.6,19.05
  Bottom 0.813: C308.1 v81.6,19.05 83.82,19.05 84.14,19.37 IC302.5
N$11  (via drill 0.3)
  Top 0.406: IC301.2 v84.77,49.21 87.31,51.75 IC301.6 | v79.69,49.21 79.69,35.88 77.47,33.66 77.47,24.45 77.79,24.13 77.79,17.14 79.06,15.88 IC302.2
  Bottom 0.406: v84.77,49.21 v79.69,49.21
  Bottom 0.61: IC302.1 IC302.2
N$15  (via drill 0.3)
  Top 0.406: v70.17,50.8 v70.17,60.64
  Bottom 0.406: IC301.5 89.85,51.44 89.22,50.8 v70.17,50.8 | v70.17,60.64 R305.1
N$16  (via drill 0.3)
  Top 0.61: v91.76,73.03 91.76,46.35 92.08,46.04 92.08,39.37 93.34,38.1 v93.34,24.13
  Bottom 0.61: T302.1 76.83,79.38 81.92,74.3 Q301.1 82.87,73.03 | Q302.1 75.25,69.22 81.6,69.22 82.87,70.48 82.87,73.03 | v91.76,73.03 82.87,73.03 | v93.34,24.13 82.23,24.13 81.6,23.5 IC302.6 IC302.7
N$17
  Top 0.61: Q301.3 80.33,76.83 76.83,73.34 Q302.2 78.42,69.22 78.42,63.82 77.79,63.18 75.88,63.18 74.61,61.91 74.61,58.74 75.25,58.1 R307.2
  Bottom 0.61: T302.2 81.92,80.64 82.87,79.69 Q301.3
N$18  (via drill 0.3)
  Top 0.61: R306.2 87.95,58.1 87.31,58.74 v87.31,75.56
  Bottom 0.61: v87.31,75.56 Q301.2
N$19  (via drill 0.3)
  Top 0.406: v87.31,39.05 IC301.3
  Top 0.61: R308.2 v66.36,51.75 63.5,51.75 63.18,51.44 63.18,43.81 66.04,40.96 C306.-
  Bottom 0.406: C306.- 78.58,39.53 79.06,39.05 v87.31,39.05 | R303.2 73.98,52.7 73.03,51.75 v66.36,51.75
N$20
  Bottom 0.61: R308.1 61.28,44.77 56.2,39.69 D306.A
N$22
  Top 0.406: R306.1 82.87,58.1 84.77,56.2 IC301.7
  Bottom 0.406: D302.C 77.79,53.66 79.06,52.39 84.14,52.39 84.77,53.02 IC301.7
N$23
  Bottom 0.406: R104.2 151.13,91.44 154.31,88.27 D101.AR
N$24
  Top 0.406: IC301.1 D303.C
N$25  (via drill 0.3)
  Top 0.406: D301.A D303.A | v94.61,43.5 v94.61,47.15
  Bottom 0.406: R302.1 68.9,43.18 69.85,42.23 88.58,42.23 D303.A v94.61,43.5 | v94.61,47.15 C301.+
N$26  (via drill 0.3)
  Top 0.406: R302.2 v68.9,48.26 | v77.15,48.26 D302.A
  Bottom 0.406: v68.9,48.26 v77.15,48.26 | R302.2 R301.1
N$27
  Bottom 0.406: R105.2 148.59,88.58 153.99,83.19 D101.AG
N$29  (via drill 0.3)
  Top 0.406: IC105.1 133.03,88.58 134.3,87.31 v134.3,74.93
  Bottom 0.406: v134.3,74.93 IC104.1
N$30  (via drill 0.3)
  Top 0.406: v133.03,72.39 v133.03,80.96
  Bottom 0.406: IC104.2 v133.03,72.39 | v133.03,80.96 IC105.4
N$32
  Bottom 0.406: OK101.3 144.78,91.44 143.51,92.71 R111.1
N$33  (via drill 0.3)
  Top 0.406: OK101.1 142.24,79.38 143.83,77.79 143.83,69.22 | 143.83,69.22 R112.2 | v143.83,66.67 143.83,69.22
  Bottom 0.406: X102.3 155.83,63.12 156.21,63.5 156.21,65.41 154.94,66.67 v143.83,66.67
N$36
  Top 1.27: R212.1 R211.1 R210.1 D208.C 134.94,15.56 133.67,16.83 133.67,22.23 | D206.C 134.94,25.72 133.67,24.45 133.67,22.23 | 133.67,22.23 OK202.4
N$37
  Bottom 1.27: OK201.2 109.22,8.89 111.12,10.79 116.52,10.79 D203.C
N$38
  Bottom 1.27: OK201.3 111.76,7.94 112.71,8.89 R201.1
N$39  (via drill 0.3)
  Top 0.61: v89.53,31.75 R202.1 | D205.C v83.82,31.75
  Bottom 0.61: L201.1 67.98,32.98 69.53,31.75 C201.1 v83.82,31.75 v89.53,31.75 | R202.1 D204.A
N$41  (via drill 0.3)
  Top 0.406: OK201.6 v111.76,17.46 | v99.38,17.46 v99.38,11.43 | v90.81,11.43 90.81,7.94 | 90.81,7.94 90.81,7.3 91.12,6.99 R203.2 | T201.2 90.49,8.26 90.81,7.94
  Bottom 0.406: v111.76,17.46 v99.38,17.46 | v99.38,11.43 v90.81,11.43
N$42  (via drill 0.3)
  Top 1.27: v143.83,4.76 143.83,18.1 144.46,18.73 D209.A
  Bottom 1.27: D207.A D209.A | Q201.E 132.08,5.71 133.03,4.76 v143.83,4.76
N$43  (via drill 0.3)
  Top 0.406: R205.2 92.08,23.81 93.03,22.86 93.03,16.51 94.3,15.24 IC201.3
  Top 0.61: D204.C v86.36,29.21 | D205.A v83.82,29.21 | v92.08,29.21 R205.2 | R206.1 v97.16,29.21
  Bottom 0.61: L201.2 67.94,27.94 68.26,27.94 69.53,29.21 C201.2 v83.82,29.21 v86.36,29.21 v92.08,29.21 v97.16,29.21
N$44
  Top 0.406: IC201.2 91.76,14.92 90.49,16.19 90.49,24.13 90.81,24.45 90.81,35.24 R202.2
  Bottom 0.406: R202.2 R204.1 R205.1
N$45
  Top 0.813: Q201.B 132.08,16.83 129.22,19.68 OK202.3
N$46
  Bottom 1.27: R212.2 R211.2 R210.2 142.56,11.43 140.65,13.34 135.25,13.34 133.35,11.43 Q201.C
N$50
  Top 0.406: OK202.1 R208.1
N$55
  Bottom 0.406: R107.2 152.4,78.42 153.35,79.38 156.37,79.38 D102.AR
N$56
  Bottom 0.406: R108.2 153.99,73.98 154.62,74.61 156.37,74.61 D102.AG
ON-P  (via drill 0.3)
  Top 0.406: R304.1 R305.2 | v122.87,73.66 v122.87,46.99 | v98.74,45.09 v98.74,59.37 | OK201.7 109.22,26.99 107.95,28.26 107.95,45.72 109.22,46.99 IC101.14
  Bottom 0.406: R108.1 141.92,73.98 141.6,73.66 v122.87,73.66 | v122.87,46.99 IC101.14 109.22,46.99 107.31,45.09 v98.74,45.09 | v98.74,59.37 81.28,59.37 R304.1
PULSE-P  (via drill 0.3)
  Top 0.406: IC101.16 112.39,41.91 113.03,41.27 v113.03,19.68 | IC201.7 v91.76,19.68
  Bottom 0.406: v113.03,19.68 OK202.2 v91.76,19.68
PWM-P  (via drill 0.3)
  Top 0.406: v114.3,38.1 v114.3,31.75 | v100.33,38.1 100.33,69.53 99.69,70.17 X101.1
  Bottom 0.406: v100.33,38.1 v114.3,38.1 | v114.3,31.75 IC101.21
SCK  (via drill 0.3)
  Top 0.406: SV101.3 115.57,80.01 116.52,79.06 v116.52,62.23 | v134.3,34.29 v134.3,60.96
  Bottom 0.406: IC101.8 v116.52,62.23 122.24,62.23 123.51,60.96 v134.3,60.96 135.57,60.96 136.84,62.23 IC104.13 | IC103.6 v134.3,34.29
SHORT-P  (via drill 0.3)
  Top 0.406: v102.87,39.37 R209.1
  Bottom 0.406: IC101.17 v102.87,39.37 88.58,39.37 87,40.96 D301.C
SPG  (via drill 0.3)
  Top 0.406: v120.97,80.01 v120.97,38.1 | v142.24,38.1 R110.1
  Bottom 0.406: R109.2 R110.1 | IC101.40 v120.97,80.01 | v120.97,38.1 v142.24,38.1
TRACK-0-E  (via drill 0.3)
  Top 1.016: X102.1 154.62,65.41 153.67,66.36 150.5,66.36 149.86,65.72 v149.86,46.04 v149.86,28.89
  Bottom 1.016: X103.1 154.56,45.15 153.67,46.04 v149.86,46.04
  Bottom 1.27: X202.1 150.02,29.05 v149.86,28.89 149.54,28.57 149.54,26.99 | 149.54,26.99 147.32,26.99 D206.A 144.15,25.72 140.97,22.54 D207.C 134.94,22.54 128.59,16.19 123.83,16.19 123.19,15.56 123.19,9.53 123.83,8.89 R201.2 | X201.1 150.5,16.83 149.54,17.78 149.54,26.99
TRACK-B-E
  Top 1.016: X202.2 151.61,23.97 151.13,24.45 151.13,44.13 | 151.13,44.13 151.13,63.82 151.45,64.14 X102.2 | X103.2 151.13,44.13
  Bottom 1.27: X202.2 157,23.97 158.43,22.54 158.43,13.65 156.53,11.75 X201.2 149.86,11.75 D208.A 144.46,15.56 141.29,18.73 D209.C 133.67,18.73 128.27,13.34 D203.A
V+
  Top 1.27: V301.IN 18.1,32.07 21.11,35.08 21.11,67.79 21.91,68.58 R312.2
  Bottom 1.27: V301.IN C304.1 22.23,20.95 D304.C 37.15,20.95 38.89,19.21 C302.+ | R312.2 25.88,69.69 26.67,70.48 57.31,70.48 57.39,70.41 | 57.39,70.41 R309.2 | Q303.1 66.99,77.79 59.69,70.48 57.47,70.48 57.39,70.41
V-  (via drill 0.3)
  Top 0.813: C305.2 46.99,13.97 v48.26,12.7
  Top 1.27: C303.- 57.78,6.67 56.2,5.08 32.23,5.08 30.16,7.14 30.16,33.02 23.65,39.53 23.65,61.12 24.45,61.91 R313.1
  Bottom 1.27: D305.A 16.83,9.05 20.64,12.7 v48.26,12.7 54.61,12.7 57.63,9.84 C303.- | R313.1 25.72,60.96 26.67,60.01 57.15,60.01 R310.1 59.37,61.91 T303.1

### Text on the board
tNames: HW: 24.05.01 | MBCAN-Projekt | (c) Dr.-Ing. Th. Wiesner | OUT | IN | B | 0 | 0 | B | L | 0 | 0 | B | mbc-93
